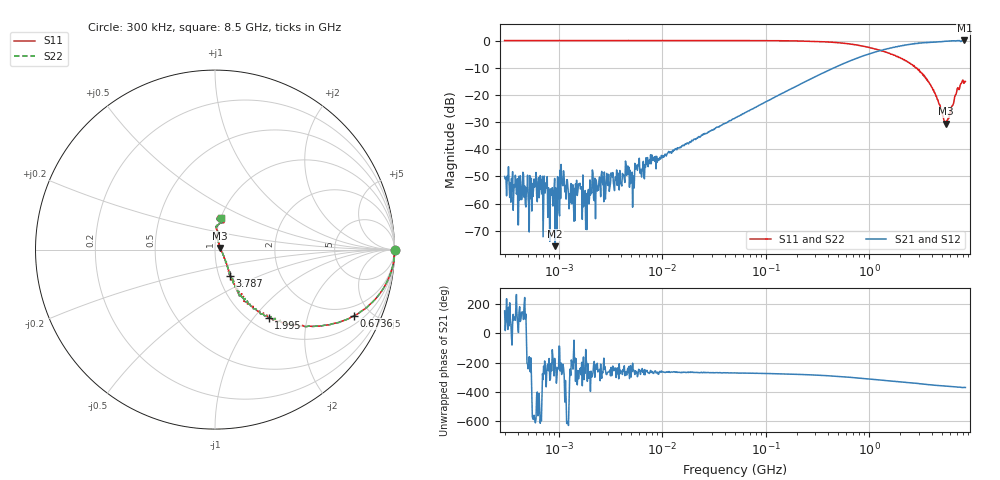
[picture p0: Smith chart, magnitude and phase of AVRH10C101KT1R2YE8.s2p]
! S-Parameter Data Generated by TDK Corporation
! Copyright(C) 2023 TDK Corporation.
! All Rights Reserved.
! TDK P/N: AVRH10C101KT1R2YE8 (Varistor)
! Property: V1mA=110V
! Size(LxWxT): 1x0.5x0.5mm
! Model Type: s2p (Touchstone File Format Version 1.0)
! Frequency: DC=Yes Start=0.3MHz Stop=8500MHz 802points Log-sweep
! Model Generated on Oct. 12, 2023
! Port Assignments:
!  1 ---N--- 2
! Applicable Conditions:
!  Temperature = 25 degC
!  DC Bias Voltage = 0 V
!  Small Signal Operation
! Terms and conditions regarding TDK Simulation Models
! (1)This simulation model is being provided solely for informational purposes. Please refer to the specifications of the products in terms of detailed characteristics of such products.
! (2)In no event shall TDK Corporation of any of its subsidiaries be liable for any loss or damage arising, directly or indirectly,
!  From any information contained in this simulation model, including, but not limited to loss or damages arising from any inaccuracies, omissions or errors in connection with such information.
! (3)Any and all copyrights on this simulation model are owned by TDK Corporation.
!  Duplication or redistribution of this simulation model without prior written permission from TDK Corporation is prohibited.
! (4)This simulation model is subject to any modification or change without any prior notice.
! (5)Neither TDK Corporation nor any of its subsidiaries shall make any warranty, express or implied,
!  Including but not limited to the correctness, implied warranties of merchantability and fitness for a particular purpose with respect to this simulation models.
! (6)The use of this simulation model shall be deemed to have consented to the terms and conditions hereof.
# Hz S MA R 50
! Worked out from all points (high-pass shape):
!   801 points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, 300 kHz to 8.5 GHz, reference 50 ohm
!   highest |S21| = 0.04 dB at 8.312 GHz (marker M1); lowest = -75.7 dB at 925.6 kHz (marker M2)
!   |S21| within 3 dB of the highest: 1.536 GHz to end of sweep
!   lowest |S11| = -30.6 dB at 5.489 GHz (marker M3), VSWR 1.06, Z = 52.9 + j1.01 ohm
!   |S11| at or under -10 dB: 2.833 GHz to end of sweep
!   |S22| runs from -30.6 to 0.0 dB; largest |S21 - S12| = 0
!   S11 on the Smith chart (normalised r, x): 300 kHz: open; 673.6 MHz: 1.41, -3.94; 1.995 GHz: 1.20, -1.20; 3.787 GHz: 1.13, -0.34; 8.5 GHz: 1.00, +0.36
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300000  1.003 -0.1  0.003155 153.3  0.003155 153.3  1.003 -0.1
413291  1.003 -0.1  0.003193 147.3  0.003193 147.3  1.003 -0.1
663333  1.001 -0.2  0.003275 105.6  0.003275 105.6  1.001 -0.2
925600  1 -0.0  0.0001647 127.4  0.0001647 127.4  1 -0.0
1080580  1.001 -0.1  0.00241 106.7  0.00241 106.7  1.001 -0.1
1404840  0.9997 0.0  0.0004742 -47.1  0.0004742 -47.1  0.9997 0.0
1667340  1.002 -0.0  0.002045 161.6  0.002045 161.6  1.002 -0.0
1779010  1 -0.1  0.001145 108.2  0.001145 108.2  1 -0.1
2573910  0.9991 -0.2  0.003355 73.6  0.003355 73.6  0.9991 -0.2
4651380  1.003 -0.2  0.004932 122.0  0.004932 122.0  1.003 -0.2
5118570  1.001 -0.2  0.003803 98.4  0.003803 98.4  1.001 -0.2
5764300  0.9982 -0.2  0.004085 63.4  0.004085 63.4  0.9982 -0.2
9160260  0.9988 -0.4  0.006637 79.8  0.006637 79.8  0.9988 -0.4
5.11488e7  1 -2.2  0.0379 89.2  0.0379 89.2  1 -2.2
2.80466e8  0.9697 -11.7  0.2022 75.6  0.2022 75.6  0.9697 -11.7
6.73562e8  0.8572 -25.5  0.4332 58.5  0.4332 58.5  0.8572 -25.5
1.54289e9  0.588 -44.4  0.7113 35.4  0.7113 35.4  0.588 -44.4
1.99538e9  0.4837 -51.8  0.7976 28.5  0.7976 28.5  0.4837 -51.8
3.78699e9  0.1686 -60.3  0.9281 9.1  0.9281 9.1  0.1686 -60.3
5.48935e9  0.02966 18.7  0.972 -0.6  0.972 -0.6  0.02966 18.7
8.31246e9  0.1687 86.5  1.004 -9.7  1.004 -9.7  0.1687 86.5
8.5e9  0.1771 79.1  0.9819 -10.2  0.9819 -10.2  0.1771 79.1
